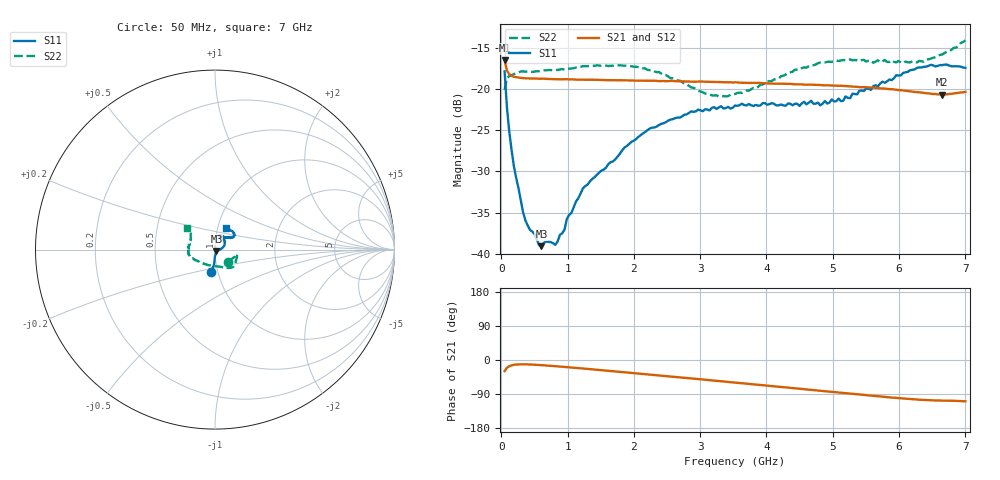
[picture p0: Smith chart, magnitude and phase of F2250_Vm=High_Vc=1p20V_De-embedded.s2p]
! Integrated Device Technology
! Corporate Headquarters
! 6024 Silver Creek Valley Road
! San Jose, CA 95138  USA
! Phone:  1-408-284-8200
! Toll Free:  1-800-223-1366
! Webpage:  http://www.idt.com/
! Timing and RF Division
! 515 Groton Road, Suite 102
! Westford, MA 01886-6024
! Device:  F2250
! Description: Voltage Variable RF Attenuator
! Frequency:  50.0 -  6000.00 MHz
! Package:  3x3 mm Thin QFN Plastic Package: 16 pin
! Ports:  2 RF, 3 DC
!  Pin  1  = GND
!  Pin  2  = NC
!  Pin  3  = RF1  = Port 1
!  Pin  4  = NC
!  Pin  5  = GND
!  Pin  6  = GND
!  Pin  7  = GND
!  Pin  8  = GND
!  Pin  9  = NC
!  Pin 10  = RF2  = Port 2
!  Pin 11  = NC
!  Pin 12  = GND
!  Pin 13  = GND
!  Pin 14  = VCNTRL
!  Pin 15  = VDD
!  Pin 16  = VMODE
! Vcntrl:  1.200 Volts
! Vmode:  +3.300 Volts
! Vdd:  +3.30  Volts
! Current:  1.331 mA
! Data:  The device was measured on a the F2250 evaluation board which has
!  individual transmission lines to the RF pins.  Data was collected
!  using a calibrated network analyzer.  The evaluation board was
!  de-embedded using a TRL calibration technique.
!  The reference plane is the edge of the package pin.
! Misc:  SN 10
!  Action Tracker AT0258
! Date Measured:  2014-11-26
! Date:  2015-10-15  MJV
! Note:
!  Integrated Device Technology supplies this data as a sample of measured
!  data at the package pin for this product.  Your particular data for this
!  product may vary.
!  Data was taken at 25 degrees C.
!  Integrated Device Technology reserves the right to change this data at anytime.
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# GHz S dB R 50
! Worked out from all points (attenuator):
!   201 points, 50 MHz to 7 GHz, reference 50 ohm
!   highest |S21| = -16.48 dB at 50 MHz (marker M1); lowest = -20.7 dB at 6.652 GHz (marker M2)
!   lowest |S11| = -39.1 dB at 606 MHz (marker M3), VSWR 1.02, Z = 50.8 - j0.758 ohm
!   |S11| at or under -10 dB: start of sweep to end of sweep
!   |S22| runs from -20.9 to -14.1 dB; largest |S21 - S12| = 0.00044
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0.05  -17.83 -99.5  -16.48 -29.2  -16.46 -29.1  -20.05 -42.0
0.08475  -22.18 -93.0  -17.75 -20.8  -17.72 -20.7  -18.69 -20.5
0.15425  -27.35 -91.6  -18.38 -14.2  -18.36 -14.1  -18.32 -12.9
0.189  -29.31 -89.0  -18.48 -12.8  -18.47 -12.8  -18.17 -12.4
0.328  -34.94 -73.7  -18.66 -11.3  -18.66 -11.3  -17.84 -12.8
0.43225  -37.09 -70.8  -18.71 -11.8  -18.68 -11.8  -17.86 -14.0
0.606  -39.08 -42.1  -18.73 -13.6  -18.71 -13.6  -17.75 -19.0
0.6755  -38.51 -38.4  -18.75 -14.4  -18.75 -14.4  -17.71 -20.4
0.8145  -38.92 -19.6  -18.78 -16.3  -18.77 -16.3  -17.68 -24.4
0.9535  -37.07 -22.8  -18.79 -18.2  -18.78 -18.3  -17.64 -28.1
0.98825  -35.79 -20.4  -18.78 -18.8  -18.78 -18.8  -17.58 -28.9
1.2315  -32.04 -5.0  -18.84 -22.4  -18.83 -22.4  -17.20 -34.1
1.857  -27.11 14.2  -18.93 -32.2  -18.90 -32.3  -17.12 -44.4
2.37825  -24.36 28.2  -19.01 -40.6  -19.00 -40.6  -17.91 -53.8
3.07325  -22.45 49.1  -19.09 -52.1  -19.08 -52.1  -20.53 -81.3
3.525  -21.99 62.2  -19.17 -59.6  -19.17 -59.7  -20.59 -112.6
4.7065  -21.76 67.5  -19.46 -79.4  -19.46 -79.4  -17.09 -162.2
5.15825  -21.40 50.7  -19.60 -87.1  -19.61 -87.1  -16.45 -171.2
5.85325  -18.82 36.0  -19.99 -98.5  -19.98 -98.6  -16.69 172.9
6.3745  -17.28 37.9  -20.45 -105.5  -20.45 -105.6  -16.64 155.2
6.6525  -17.07 44.6  -20.65 -107.1  -20.66 -107.2  -15.78 145.8
7  -17.41 62.1  -20.32 -109.1  -20.33 -109.2  -14.08 142.0
